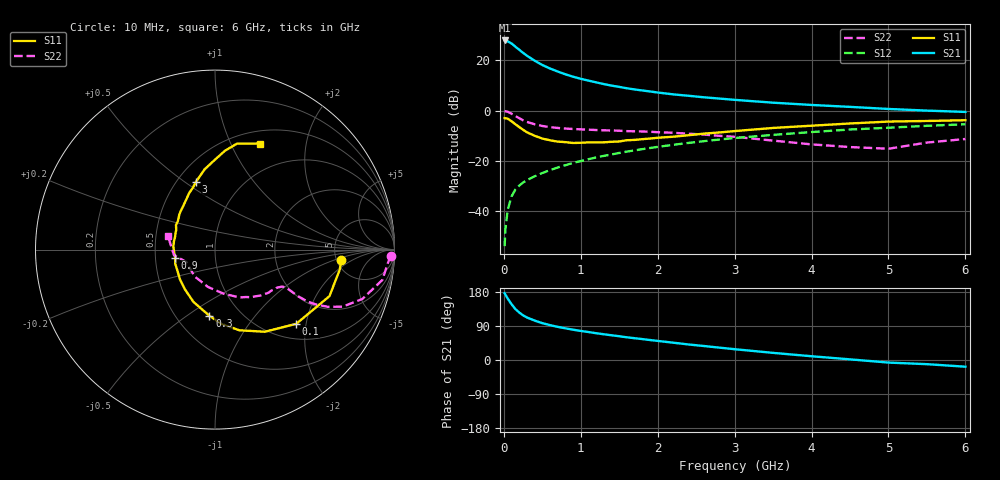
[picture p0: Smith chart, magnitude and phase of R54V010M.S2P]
! SIEMENS Small Signal Semiconductors
! BFR183
! Si NPN RF Bipolar Junction Transistor in SOT23
! VCE = 4 V  IC = 10 mA
! Common Emitter S-Parameters:  May  1996
# GHz  S  MA  R  50
!  f  S11  S21  S12  S22
! GHz  MAG  ANG  MAG  ANG  MAG  ANG  MAG  ANG
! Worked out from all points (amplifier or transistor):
!   36 points, 10 MHz to 6 GHz, reference 50 ohm
!   highest |S21| = 27.9 dB at 10 MHz (marker M1)
!   |S21| within 3 dB of that: start of sweep to 171.6 MHz
!   unconditionally stable (mu >= 1): 777.2 MHz to 2.484 GHz
!   at 250 MHz: K = 0.62, MSG = 25.8 dB, |S12| = -28.6 dB
!   at 1.4 GHz: K = 1.06, MAG = 12.3 dB, |S12| = -17.5 dB
!   at 6 GHz: K = 0.89, MSG = 2.5 dB, |S12| = -5.5 dB
!   lowest NFmin = 1.30 dB at 450 MHz
!   S11 on the Smith chart (normalised r, x): 10 MHz: 5.50, -1.30; 100 MHz: 1.33, -1.76; 300 MHz: 0.72, -0.61; 900 MHz: 0.63, -0.06; 3 GHz: 0.62, +0.55; 6 GHz: 0.65, +1.30
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0.01  0.7065 -4.8  24.84 176.3  0.002 86.1  0.9809 -2.0
0.02  0.7039 -9.1  24.55 172.5  0.0043 89.0  0.9669 -4.3
0.05  0.6886 -22.1  23.89 162.3  0.0105 80.4  0.9474 -10.3
0.1  0.6132 -42.4  21.63 147.1  0.0196 73.7  0.8661 -18.5
0.15  0.535 -58.8  18.68 134.5  0.0268 67.0  0.7788 -24.1
0.2  0.4696 -73.2  16.24 125.3  0.0321 64.6  0.705 -26.9
0.25  0.4143 -85.4  14.09 117.8  0.037 62.8  0.6409 -28.5
0.3  0.3696 -94.9  12.36 112.2  0.0412 62.9  0.5948 -29.3
0.4  0.3152 -112.4  9.835 104.1  0.0491 62.7  0.5337 -29.3
0.5  0.2774 -127.2  8.069 97.3  0.0571 63.8  0.4932 -28.8
0.6  0.2559 -139.8  6.873 92.0  0.0652 64.7  0.468 -28.4
0.7  0.2409 -149.8  5.984 87.5  0.0736 65.5  0.451 -28.4
0.9  0.2261 -168.7  4.713 80.0  0.0907 65.6  0.4295 -28.7
1.1  0.2327 175.6  3.943 73.8  0.1078 65.6  0.4163 -30.2
1.3  0.2334 162.6  3.364 67.9  0.1254 64.8  0.4045 -31.8
1.6  0.2568 147.9  2.776 59.9  0.1526 63.0  0.3897 -35.6
2.2  0.3015 125.8  2.102 45.7  0.2079 58.3  0.3613 -45.0
3  0.3903 106.0  1.634 28.5  0.2838 49.8  0.3003 -62.6
3.5  0.4508 97.4  1.435 18.8  0.3279 43.6  0.2523 -78.2
4.5  0.5531 84.3  1.184 1.7  0.4199 31.4  0.1877 -127.3
5.5  0.6204 72.0  0.998 -11.0  0.4971 19.5  0.2307 -172.2
6  0.6425 66.9  0.939 -17.7  0.5335 11.8  0.2717 164.3
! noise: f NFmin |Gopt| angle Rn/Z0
0.45  1.3  0.15  45  0.18
0.9  1.4  0.2  125  0.19
1.8  2.1  0.34  -170  0.14
